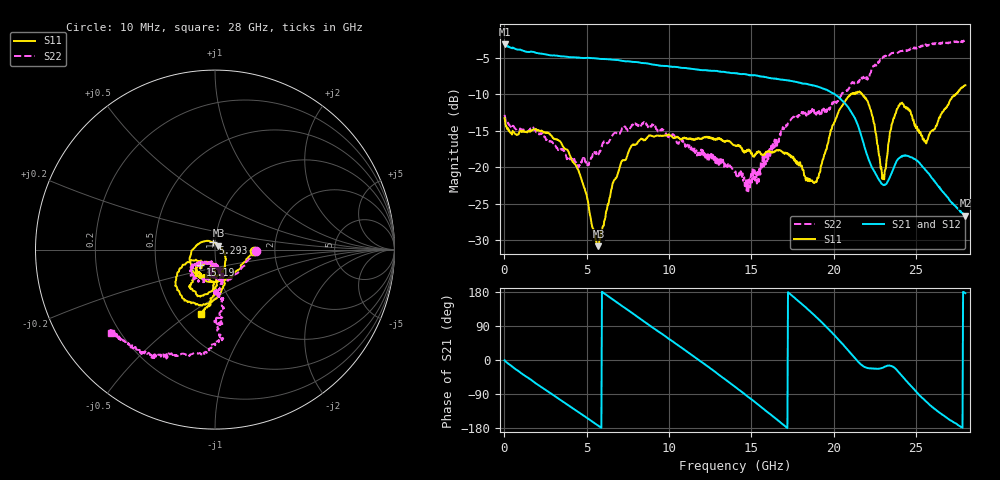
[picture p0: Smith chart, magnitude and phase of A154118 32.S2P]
!  2-Port S-parameters saved by WinCal
! VAR MeasName=S-Parameters (CALIBRATED_DATA) read from VNA (N5230A)
! VAR MeasDate=2015-9-10 14:36:46
! VAR NAME=A154118 32
! VAR FILENAME=A154118 32.S2P
! VAR DATE=2015-9-10 14:36:46
! VAR PHYS_PORTS=1,2
# Hz S DB R 50
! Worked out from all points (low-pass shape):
!   801 points, 10 MHz to 28 GHz, reference 50 ohm
!   highest |S21| = -3.13 dB at 10 MHz (marker M1); lowest = -26.6 dB at 28 GHz (marker M2)
!   |S21| within 3 dB of the highest: start of sweep to 9.949 GHz
!   lowest |S11| = -30.8 dB at 5.713 GHz (marker M3), VSWR 1.06, Z = 51.9 + j2.25 ohm
!   |S11| at or under -10 dB: start of sweep to 21.03 GHz; 21.74 GHz to 27.39 GHz (5.65 GHz wide, 23 % of centre); 27.4389 GHz to 27.44063 GHz (1.73 MHz wide, 0.0063 % of centre)
!   |S22| runs from -23.3 to -2.6 dB; largest |S21 - S12| = 0.0078
!   S11 on the Smith chart (normalised r, x): 10 MHz: 1.55, -0.03; 5.293 GHz: 0.98, +0.08; 15.19 GHz: 0.83, -0.14; 28 GHz: 0.67, -0.55
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1e7  -13.25 -2.6  -3.13 -0.7  -3.19 -0.8  -12.81 -2.0
1.094612e9  -14.95 -65.0  -3.96 -37.3  -3.99 -37.2  -14.82 -44.7
2.319175e9  -15.08 -121.2  -4.45 -73.8  -4.45 -73.6  -15.55 -84.8
4.698325e9  -21.77 148.0  -5.00 -143.4  -4.98 -143.5  -19.32 -104.1
5.293112e9  -27.74 104.8  -5.03 -161.2  -5.02 -161.3  -18.67 -98.7
5.712962e9  -30.80 48.8  -5.10 -174.0  -5.07 -174.0  -18.22 -94.3
7.112462e9  -19.18 -59.4  -5.38 143.4  -5.36 143.3  -14.88 -111.3
9.351662e9  -15.64 -109.9  -6.04 75.1  -5.98 74.9  -14.99 -137.9
1.166084e10  -16.12 -125.9  -6.57 4.3  -6.53 3.8  -17.65 -139.1
1.4005e10  -17.00 -137.0  -7.11 -70.6  -7.08 -71.1  -20.61 -130.9
1.519458e10  -18.43 -134.9  -7.36 -110.1  -7.36 -110.8  -20.38 -84.7
1.701392e10  -18.15 -129.8  -8.04 -173.3  -8.04 -174.0  -14.30 -78.1
1.869332e10  -21.79 -105.9  -8.72 123.4  -8.78 123.1  -11.98 -88.8
1.974295e10  -15.74 -73.5  -9.57 78.9  -9.50 78.2  -12.08 -84.5
2.110746e10  -9.93 -104.8  -12.56 14.3  -12.55 13.3  -8.34 -85.1
2.21221e10  -11.38 -143.2  -18.91 -21.8  -18.92 -23.0  -7.51 -85.9
2.29618e10  -21.60 -123.5  -22.31 -20.7  -22.43 -21.7  -5.05 -94.0
2.334666e10  -16.48 -86.6  -21.67 -14.9  -21.67 -15.4  -4.66 -99.8
2.397644e10  -11.54 -105.1  -18.73 -33.5  -18.77 -34.4  -4.16 -108.9
2.467619e10  -12.44 -124.2  -18.62 -67.7  -18.68 -69.0  -3.69 -114.4
2.558586e10  -16.46 -107.9  -20.40 -108.3  -20.43 -108.2  -3.12 -120.5
2.8e10  -8.74 -102.6  -26.64 176.5  -26.56 176.1  -2.60 -141.1
